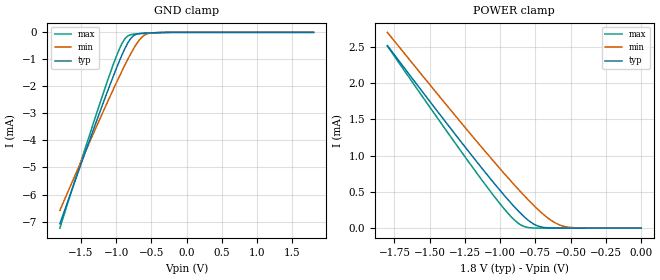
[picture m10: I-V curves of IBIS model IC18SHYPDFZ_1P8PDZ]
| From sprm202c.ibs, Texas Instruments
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|   Model IC18SHYPDFZ_1P8PDZ
[Model]   IC18SHYPDFZ_1P8PDZ
Model_type   Input
Polarity   Non-Inverting
Vinl =   0.8400V
Vinh =   0.9800V
C_comp   0.8000pF   0.9300pF   0.6600pF
[Model Spec]
|   typ   min   max
Vinh   0.98V   0.86V   1.05V
Vinl   0.84V   0.70V   0.91V
[Temperature Range]   25.0000   0.1250k   -40.0000
[Voltage Range]   1.8000V   1.6200V   1.9500V
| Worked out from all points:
|   GND clamp passes 1 mA (typ) near -0.95 V on its own axis
|   POWER clamp passes 1 mA (typ) near -1.20 V on its own axis
[GND_clamp]
| voltage   I(typ)   I(min)   I(max)
-1.8V     -7.086mA   -6.588mA   -7.245mA
-1.36V    -3.86mA    -3.954mA   -3.645mA
-1.08V    -1.881mA   -2.326mA   -1.462mA
-1V       -1.344mA   -1.875mA   -894.8uA
-920mV    -840.7uA   -1.437mA   -418.3uA
-880mV    -611.6uA   -1.224mA   -243.5uA
-840mV    -408.5uA   -1.017mA   -137.6uA
-760mV    -131.4uA   -629.6uA   -69.8uA
-680mV    -46.27uA   -305.8uA   -50.18uA
-600mV    -28.37uA   -100.7uA   -36.79uA
-520mV    -19.25uA   -27.87uA   -24.83uA
1.8V      2.484nA    6.669nA    4.54nA
[POWER_clamp]
| voltage   I(typ)   I(min)   I(max)
-1.8V     2.515mA    2.698mA    2.51mA
-1.4V     1.497mA    1.743mA    1.394mA
-1.12V    803.4uA    1.089mA    638.5uA
-960mV    427.4uA    728.5uA    240uA
-900mV    296.1uA    597.6uA    114.6uA
-860mV    214.4uA    512.3uA    51.52uA
-820mV    140.4uA    429.2uA    16uA
-740mV    35.44uA    272.5uA    673.8nA
-640mV    2.083uA    109.8uA    10.78nA
-560mV    119.4nA    32.17uA    5.014nA
-440mV    3.921nA    2.344uA    4.775nA
0V        2.484nA    4.87nA     4.588nA
